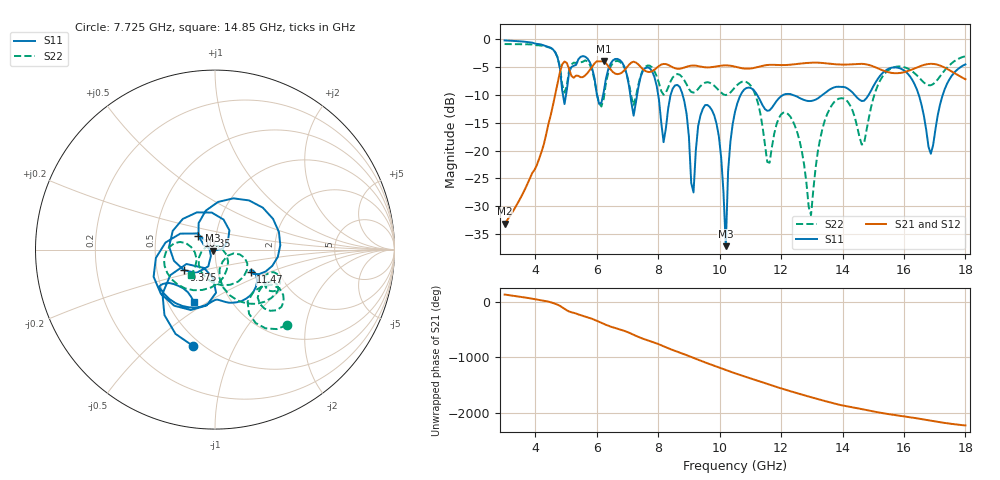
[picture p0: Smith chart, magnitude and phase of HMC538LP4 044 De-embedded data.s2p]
! Chelmsford, MA 01824
! http://www.hittite.com
! Tel: 978-250-3343
! Fax: 978-250-3373
! Device  :  HMC538LP4
! Description:  600 Analog Phase Shifter
! Frequency  :  6.0 GHz - 15.0 GHz
! Package  :  LP4  - 4x4 mm Quad Flatpack No-Lead (QFN) Plastic Package: 24 pin
! Ports  :  2 RF, 1 DC
!  Pin  3  = Rfin  = Port 1
!  Pin  16  = Rfout = Port 2
!  pin  21  = vCTL
! Voltages:  VCTL  = 0 to 5.0 Volts
! Currents :  Vb(V)  Vd(V)  Ib(mA)  Id(mA)
!  0.00  4.40  0.000000	0.479475
! Data:  The device was measured on evaluation board 111296-1.
!  Data was collected using a calibrated network analyzer.
!  The evaluation circuit board was modeled and simulated.This was use
!  to removed the evaluation board circuit from the measured data.
!  The reference plane is the center of the package pin.
! Misc:  Lot #
!Date Measured:  03 - 11 -2009
! Date:  03 - 17 -2009
! Note:
!  Hittite Microwave supplies this data as a sample of measured data at the
!  package pin for this package product.  Your particular data for this product
!  may vary.
!  Data was taken at 25 degrees C.
!  Hittite Microwave reserves the right to change this data at anytime.
# MHz S MA R 50
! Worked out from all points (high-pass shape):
!   201 points, 3 GHz to 18 GHz, reference 50 ohm
!   highest |S21| = -3.91 dB at 6.225 GHz (marker M1); lowest = -33.2 dB at 3 GHz (marker M2)
!   |S21| within 3 dB of the highest: 4.762 GHz to 17.91 GHz (13.15 GHz wide, 116 % of centre)
!   lowest |S11| = -37.2 dB at 10.2 GHz (marker M3), VSWR 1.03, Z = 48.8 - j0.647 ohm
!   |S11| at or under -10 dB: 8.796 GHz to 10.68 GHz (1.887 GHz wide, 19.4 % of centre); 11.22 GHz to 12.06 GHz (839.2 MHz wide, 7.21 % of centre); 12.39 GHz to 13.34 GHz (948.1 MHz wide, 7.37 % of centre)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
!   |S22| runs from -31.6 to -0.8 dB; largest |S21 - S12| = 0.0023
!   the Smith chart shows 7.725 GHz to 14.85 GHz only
!   S11 on the Smith chart (normalised r, x): 7.725 GHz: 0.45, -0.69; 9.375 GHz: 0.69, -0.17; 10.35 GHz: 0.82, +0.13; 11.47 GHz: 1.44, -0.39; 14.85 GHz: 0.68, -0.44
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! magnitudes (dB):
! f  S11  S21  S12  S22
! 3 GHz  -0.2  -33.2  -33.2  -0.8
! 4.95 GHz  -11.6  -4.0  -4.0  -9.5
! 5.55 GHz  -3.0  -6.8  -6.8  -4.0
! 6.225 GHz  -9.5  -3.9  -3.9  -10.7
! 7.725 GHz  -5.2  -5.9  -5.9  -4.7
! 8.025 GHz  -10.8  -4.8  -4.8  -7.8
! 8.175 GHz  -18.5  -4.4  -4.4  -10.0
! 8.775 GHz  -9.6  -5.2  -5.2  -6.8
! 9.15 GHz  -27.5  -4.7  -4.7  -9.6
! 9.375 GHz  -13.7  -4.9  -4.9  -8.4
! 9.9 GHz  -15.2  -4.9  -4.9  -8.7
! 10.2 GHz  -37.2  -4.7  -4.7  -10.0
! 10.35 GHz  -18.5  -4.7  -4.7  -9.5
! 10.5 GHz  -13.0  -4.9  -4.9  -8.6
! 11.47 GHz  -12.5  -4.7  -4.7  -19.0
! 12.22 GHz  -9.8  -4.6  -4.6  -13.4
! 13.05 GHz  -11.0  -4.2  -4.2  -27.0
! 13.72 GHz  -8.6  -4.4  -4.5  -11.3
! 14.85 GHz  -10.0  -4.6  -4.6  -14.3
! 15.53 GHz  -5.2  -5.9  -6.0  -5.4
! 16.88 GHz  -20.6  -4.4  -4.4  -8.2
! 18 GHz  -4.5  -7.2  -7.2  -3.0
